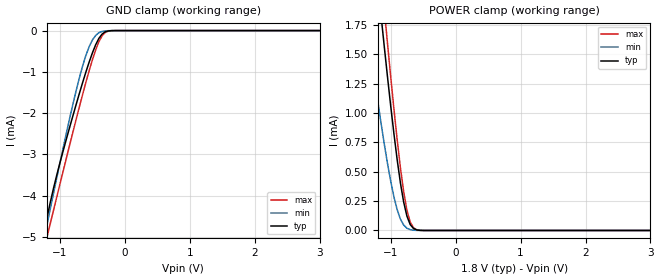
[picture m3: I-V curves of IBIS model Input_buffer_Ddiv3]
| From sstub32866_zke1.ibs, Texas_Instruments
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|   Model   Input_buffer_Ddiv3
[Model]   Input_buffer_Ddiv3
Model_type   Input
Polarity   Non-Inverting
Vinl   =   0.650V
Vinh   =   1.150V
|Variable   typ   min   max
C_comp   1.315e-13   1.291e-13   2.035e-13
|Variable   typ   min   max
[Voltage range]   1.8   1.7   1.9
|Variable   typ   min   max
[Temperature range]  27   125   0.0
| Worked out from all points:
|   GND clamp passes 1 mA (typ) near -0.60 V on its own axis
|   POWER clamp passes 1 mA (typ) near -0.99 V on its own axis
[GND_clamp]
|Volts   typ   min   max
-3.6V     -27.11mA   -23.87mA   -28.31mA
-1.25V    -4.934mA   -5.104mA   -5.35mA
-1.2V     -4.545mA   -4.72mA    -5.017mA
-1.15V    -4.179mA   -4.339mA   -4.691mA
-1.05V    -3.515mA   -3.585mA   -4.047mA
-850mV    -2.347mA   -2.132mA   -2.777mA
-650mV    -1.261mA   -858.5uA   -1.549mA
-500mV    -544uA     -230.5uA   -712.1uA
-400mV    -190.8uA   -52.58uA   -272.2uA
-300mV    -28.67uA   -6.928uA   -43.39uA
-200mV    -1.717uA   -638.4nA   -2.134uA
3.6V      0A         0A         0A
[POWER_clamp]
|Volts   typ   min   max
-3.6V     16.04mA    11.77mA    17.89mA
-1.35V    2.945mA    1.699mA    3.437mA
-1.15V    1.839mA    919uA      2.196mA
-1.1V     1.573mA    740.6uA    1.894mA
-1.05V    1.313mA    573uA      1.598mA
-950mV    823uA      285.7uA    1.033mA
-850mV    404.1uA    96.12uA    534.1uA
-750mV    122uA      19.2uA     173uA
-700mV    50.7uA     7.284uA    73.17uA
-650mV    17.19uA    2.559uA    24.32uA
-500mV    265.9nA    0A         251.8nA
3.6V      0A         0A         0A
